(* Logix 5000 AddOnInstructionDefinition export YAI_Assy_72_73_101_EIP_Hz; software revision 17.00 *)

ADD_ON_INSTRUCTION YAI_Assy_72_73_101_EIP_Hz   (* revision 1.0, vendor Yaskawa America, Inc. *)
// YAI Assembly 72/73 and 101
// Speed is given in Hz
// Torque is given in % rated torque
// Help:
// This add-on instruction is for use with input assemblie 72 or 73 and output assemblies 22 or 23.
// Node_Input_Assy is defined as the node's input assembly integer array.
// Node_Output_Assy is defined as the node's output assembly integer array.
// Torque limit/reference and torque output variables are only available with A1000.
VAR_IN_OUT
   Node_Input_Assy : AB:ETHERNET_MODULE_INT_6Bytes:I:0; {required}   // Input assembly words
   Node_Output_Assy : AB:ETHERNET_MODULE_INT_8Bytes:O:0; {required}   // Output assembly words
END_VAR
VAR_INPUT
   RunFwd : BOOL; {visible}   // Forward run command
   RunRev : BOOL; {visible}   // Reverse run command
   FaultReset : BOOL; {visible}   // Fault reset command
   Net_Control : BOOL;   // Network control bit to switch between b1-02 setting and network.
   Net_Ref : BOOL;   // Network reference bit to switch between b1-01 setting and network.
   Freq_Ref : REAL; {visible}   // Frequency reference command in Hz (xx.xx resolution)
   Torq_Ref_Limit : REAL; {visible}   // Torque reference/limit (A1000 only) Engineering Units
END_VAR
VAR_OUTPUT
   Faulted : BOOL; {visible}   // Drive faulted status bit
   Warning : BOOL; {visible}   // Drive warning (alarm) status bit
   RunningFwd : BOOL; {visible}   // Drive running forward status bit
   RunningRev : BOOL; {visible}   // Drive running reverse status bit
   Ready : BOOL; {visible}   // Drive ready status bit
   NetRefStatus : BOOL; {visible}   // Drive network reference status bit (1 = reference coming from network)
   NetCtrlStatus : BOOL; {visible}   // Drive network run source status bit (1 = source coming from network)
   Drive_State : INT;   // Drive Status - Refer to class 0x29, Instance 0x1, Attribute 0x6 for details
   At_Speed : BOOL; {visible}   // Drive at commanded speed status bit
   Output_Freq : REAL; {visible}   // Drive output frequency in Hz (xx.xx resolution)
   Torque_Actual : REAL; {visible}   // Drive torque output in engineering units.
END_VAR
VAR_INPUT
   Motor_Rated_Torq : REAL := 100.0; {visible}   // Motor rated torque (Engineering units)
   MFI_3 : BOOL;
   MFI_4 : BOOL;
   MFI_5 : BOOL;
   MFI_6 : BOOL;
   MFI_7 : BOOL;
   MFI_8 : BOOL;
   External_Fault : BOOL;
   MFO_1 : BOOL;
   MFO_2 : BOOL;
   MFO_3 : BOOL;
   Torq_Comp : REAL;
END_VAR
VAR
   FRef_Convert : DINT;
   FOut_Convert : REAL;
   FOut_Temp : REAL;
   TRef_Convert : INT;
   DriveStatusTempBits : INT;
   TOut_Convert : REAL;
   TOut_Temp : REAL;
   Motor_Torq_Temp : REAL;
   Tout_Convert_Temp : REAL;
   TComp_Convert : INT;
END_VAR

ROUTINE Logic   (* ladder *)
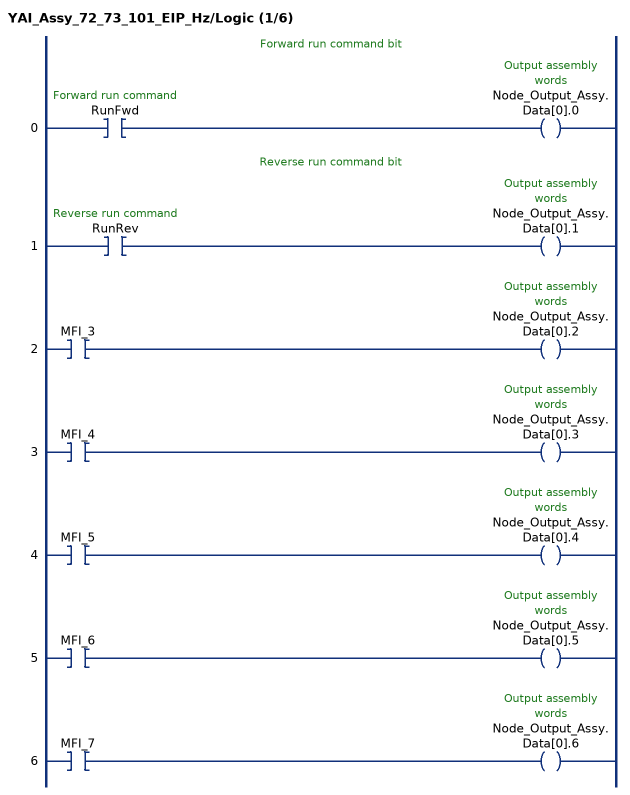
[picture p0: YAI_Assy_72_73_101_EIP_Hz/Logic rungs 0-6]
   // Forward run command bit
   0: XIC(RunFwd)OTE(Node_Output_Assy.Data[0].0);
   // Reverse run command bit
   1: XIC(RunRev)OTE(Node_Output_Assy.Data[0].1);
   2: XIC(MFI_3)OTE(Node_Output_Assy.Data[0].2);
   3: XIC(MFI_4)OTE(Node_Output_Assy.Data[0].3);
   4: XIC(MFI_5)OTE(Node_Output_Assy.Data[0].4);
   5: XIC(MFI_6)OTE(Node_Output_Assy.Data[0].5);
   6: XIC(MFI_7)OTE(Node_Output_Assy.Data[0].6);
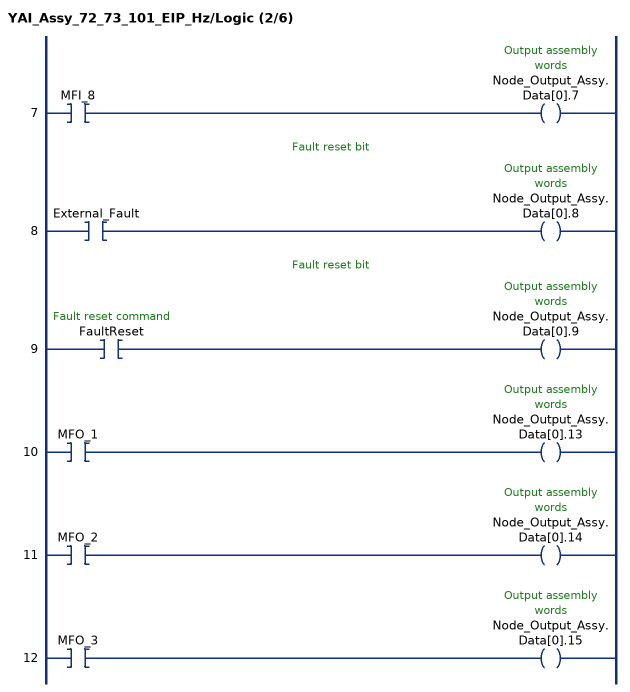
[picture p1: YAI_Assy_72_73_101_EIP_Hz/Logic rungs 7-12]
   7: XIC(MFI_8)OTE(Node_Output_Assy.Data[0].7);
   // Fault reset bit
   8: XIC(External_Fault)OTE(Node_Output_Assy.Data[0].8);
   // Fault reset bit
   9: XIC(FaultReset)OTE(Node_Output_Assy.Data[0].9);
   10: XIC(MFO_1)OTE(Node_Output_Assy.Data[0].13);
   11: XIC(MFO_2)OTE(Node_Output_Assy.Data[0].14);
   12: XIC(MFO_3)OTE(Node_Output_Assy.Data[0].15);
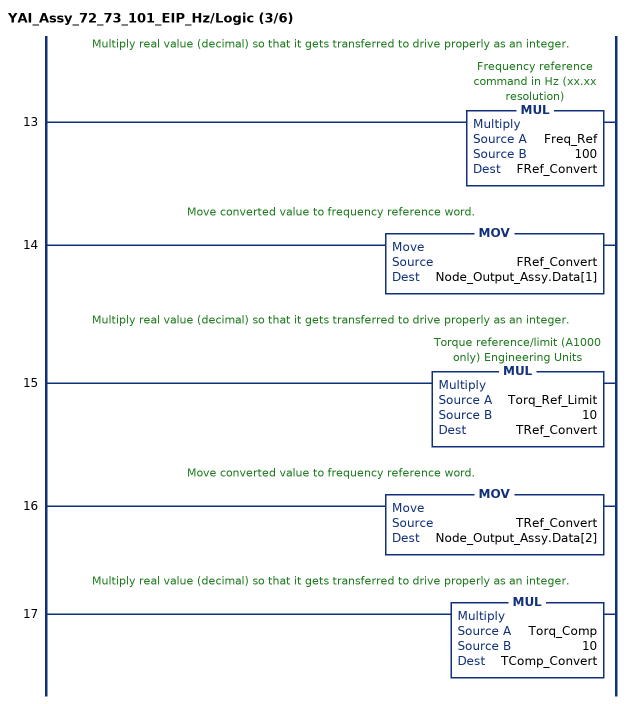
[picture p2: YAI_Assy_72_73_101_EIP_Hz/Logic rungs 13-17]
   // Multiply real value (decimal) so that it gets transferred to drive properly as an integer.
   13: MUL(Freq_Ref,100,FRef_Convert);
   // Move converted value to frequency reference word.
   14: MOV(FRef_Convert,Node_Output_Assy.Data[1]);
   // Multiply real value (decimal) so that it gets transferred to drive properly as an integer.
   15: MUL(Torq_Ref_Limit,10,TRef_Convert);
   // Move converted value to frequency reference word.
   16: MOV(TRef_Convert,Node_Output_Assy.Data[2]);
   // Multiply real value (decimal) so that it gets transferred to drive properly as an integer.
   17: MUL(Torq_Comp,10,TComp_Convert);
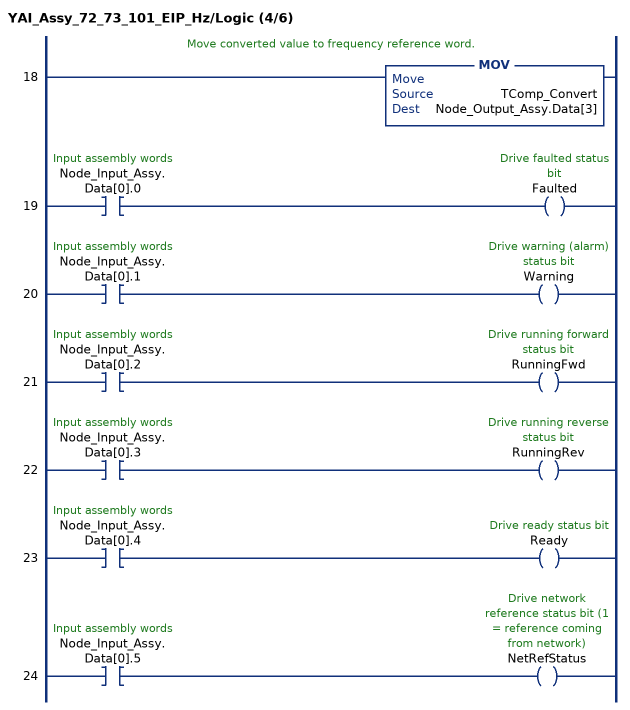
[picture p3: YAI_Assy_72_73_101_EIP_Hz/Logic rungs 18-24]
   // Move converted value to frequency reference word.
   18: MOV(TComp_Convert,Node_Output_Assy.Data[3]);
   19: XIC(Node_Input_Assy.Data[0].0)OTE(Faulted);
   20: XIC(Node_Input_Assy.Data[0].1)OTE(Warning);
   21: XIC(Node_Input_Assy.Data[0].2)OTE(RunningFwd);
   22: XIC(Node_Input_Assy.Data[0].3)OTE(RunningRev);
   23: XIC(Node_Input_Assy.Data[0].4)OTE(Ready);
   24: XIC(Node_Input_Assy.Data[0].5)OTE(NetRefStatus);
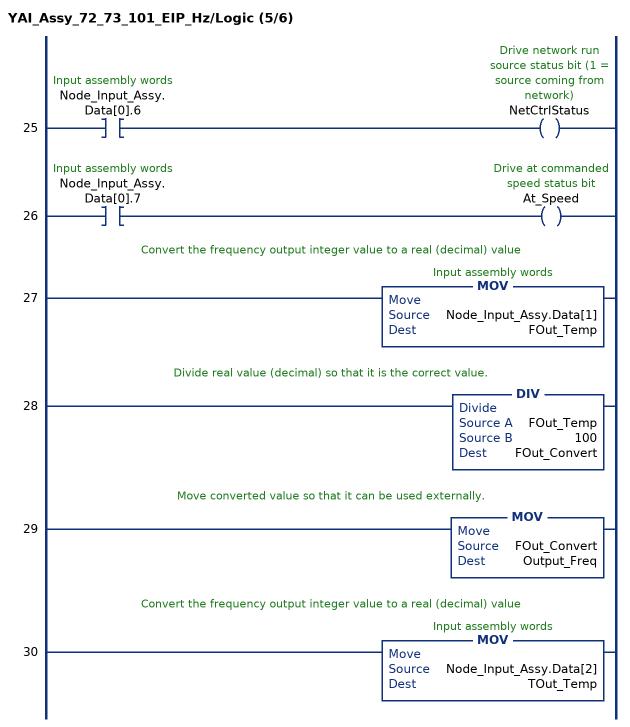
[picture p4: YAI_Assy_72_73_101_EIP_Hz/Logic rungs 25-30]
   25: XIC(Node_Input_Assy.Data[0].6)OTE(NetCtrlStatus);
   26: XIC(Node_Input_Assy.Data[0].7)OTE(At_Speed);
   // Convert the frequency output integer value to a real (decimal) value
   27: MOV(Node_Input_Assy.Data[1],FOut_Temp);
   // Divide real value (decimal) so that it is the correct value.
   28: DIV(FOut_Temp,100,FOut_Convert);
   // Move converted value so that it can be used externally.
   29: MOV(FOut_Convert,Output_Freq);
   // Convert the frequency output integer value to a real (decimal) value
   30: MOV(Node_Input_Assy.Data[2],TOut_Temp);
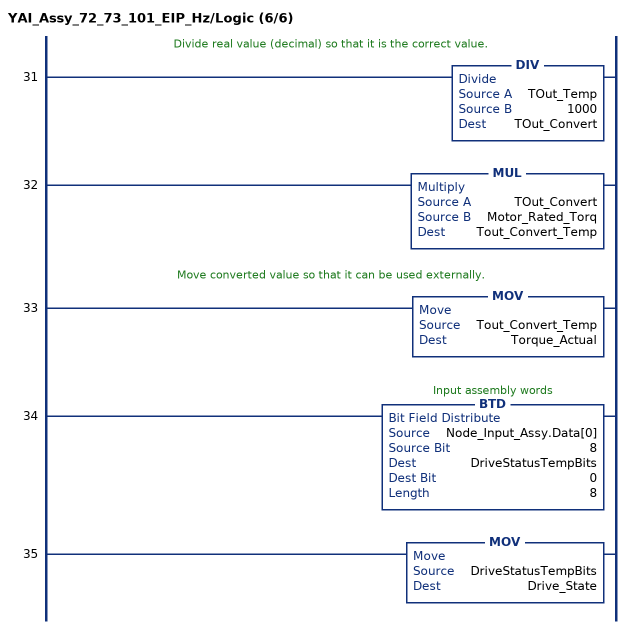
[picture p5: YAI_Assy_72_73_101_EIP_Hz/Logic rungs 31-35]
   // Divide real value (decimal) so that it is the correct value.
   31: DIV(TOut_Temp,1000,TOut_Convert);
   32: MUL(TOut_Convert,Motor_Rated_Torq,Tout_Convert_Temp);
   // Move converted value so that it can be used externally.
   33: MOV(Tout_Convert_Temp,Torque_Actual);
   34: BTD(Node_Input_Assy.Data[0],8,DriveStatusTempBits,0,8);
   35: MOV(DriveStatusTempBits,Drive_State);
END_ROUTINE
END_ADD_ON_INSTRUCTION
